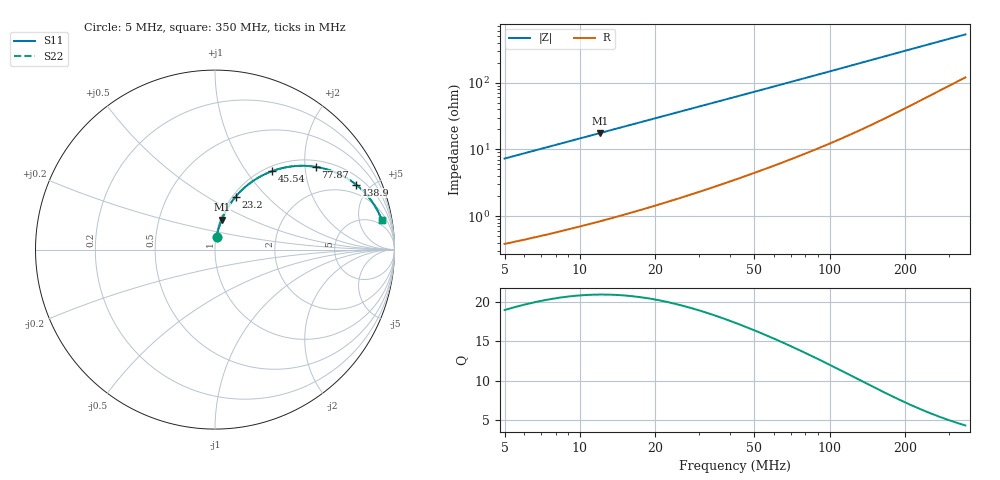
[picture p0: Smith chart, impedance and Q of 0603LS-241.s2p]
# MHz S MA R 50
!Freq  MagS11  AngS11  MagS21  AngS21  MagS12  AngS12  MagS22  AngS22
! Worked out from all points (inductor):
!   801 points, 5 MHz to 350 MHz, reference 50 ohm
!   read as one part in series: L = 232 nH near 5.107 MHz
!   highest Q = 21 at 12.01 MHz (marker M1), where L = 232 nH
!   S11 on the Smith chart (normalised r, x): 5 MHz: 1.01, +0.15; 23.2 MHz: 1.03, +0.68; 45.54 MHz: 1.08, +1.33; 77.87 MHz: 1.17, +2.28; 138.9 MHz: 1.42, +4.10; 350 MHz: 3, +10
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5  0.07242 82.8  0.9936 -4.1  0.9936 -4.1  0.07242 82.8
6.486079  0.09368 81.8  0.9909 -5.4  0.9909 -5.4  0.09368 81.8
8.06387  0.1161 80.6  0.9876 -6.7  0.9876 -6.7  0.1161 80.6
9.919552  0.1421 79.1  0.9831 -8.2  0.9831 -8.2  0.1421 79.1
12.0094  0.171 77.4  0.9772 -9.8  0.9772 -9.8  0.171 77.4
14.38594  0.2032 75.5  0.9695 -11.7  0.9695 -11.7  0.2032 75.5
17.05069  0.2385 73.5  0.9597 -13.8  0.9597 -13.8  0.2385 73.5
23.20127  0.3156 68.8  0.9332 -18.4  0.9332 -18.4  0.3156 68.8
27.94053  0.3706 65.3  0.9098 -21.7  0.9098 -21.7  0.3706 65.3
33.11606  0.426 61.7  0.8821 -25.2  0.8821 -25.2  0.426 61.7
39.04237  0.4834 57.9  0.8486 -28.9  0.8486 -28.9  0.4834 57.9
45.54293  0.5392 54.1  0.811 -32.6  0.811 -32.6  0.5392 54.1
53.69311  0.5994 49.7  0.7639 -36.7  0.7639 -36.7  0.5994 49.7
62.63302  0.6544 45.4  0.7141 -40.8  0.7141 -40.8  0.6544 45.4
77.869  0.7265 39.4  0.6363 -46.4  0.6363 -46.4  0.7265 39.4
97.845  0.7915 33.2  0.5497 -52.1  0.5497 -52.1  0.7915 33.2
120.3614  0.8391 28.0  0.4717 -56.7  0.4717 -56.7  0.8391 28.0
138.9182  0.8655 24.7  0.4201 -59.4  0.4201 -59.4  0.8655 24.7
178.303  0.9001 19.6  0.3381 -63.3  0.3381 -63.3  0.9001 19.6
235.012  0.9248 15.0  0.2617 -66.0  0.2617 -66.0  0.9248 15.0
293.7364  0.9373 12.0  0.2116 -66.9  0.2116 -66.9  0.9373 12.0
350  0.944 10.0  0.1789 -66.8  0.1789 -66.8  0.944 10.0
